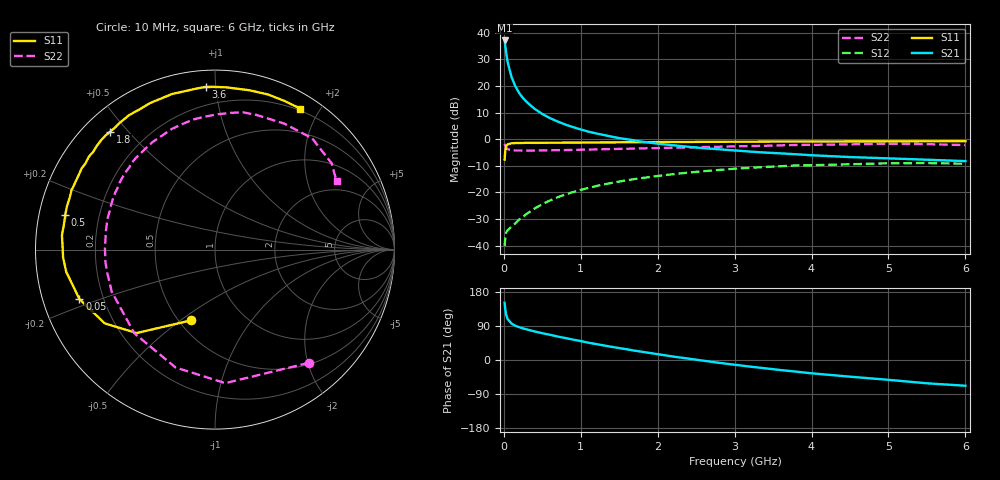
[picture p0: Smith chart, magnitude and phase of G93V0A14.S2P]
! SIEMENS Small Signal Semiconductors
! BFG235
! Si NPN RF Bipolar Junction Transistor in SOT223
! VCE = 3 V  IC = 140 mA
! Common Emitter S-Parameters:  July  1994
# GHz  S  MA  R  50
!  f  S11  S21  S12  S22
! GHz  MAG  ANG  MAG  ANG  MAG  ANG  MAG  ANG
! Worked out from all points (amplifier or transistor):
!   40 points, 10 MHz to 6 GHz, reference 50 ohm
!   highest |S21| = 37.1 dB at 10 MHz (marker M1)
!   |S21| within 3 dB of that: start of sweep to 23.17 MHz
!   unconditionally stable (mu >= 1): 443.8 MHz to 1.532 GHz
!   at 200 MHz: K = 0.81, MSG = 23.7 dB, |S12| = -30.1 dB
!   at 1.5 GHz: K = 1.00, MAG = 7.8 dB, |S12| = -15.9 dB
!   at 6 GHz: K = 0.91, MSG = 0.5 dB, |S12| = -9.2 dB
!   S11 on the Smith chart (normalised r, x): 10 MHz: 0.58, -0.55; 50 MHz: 0.11, -0.18; 500 MHz: 0.08, +0.11; 1.8 GHz: 0.08, +0.45; 3.6 GHz: 0.09, +0.94; 6 GHz: 0.18, +1.76
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0.01  0.4154 -108.5  71.63 150.7  0.0098 61.2  0.8197 -50.3
0.02  0.6378 -133.2  55.05 131.3  0.0147 46.4  0.7462 -85.6
0.03  0.739 -146.2  42.51 119.6  0.0177 39.7  0.6926 -108.5
0.05  0.804 -159.9  27.95 107.7  0.0195 32.5  0.6476 -134.0
0.1  0.8381 -171.5  14.66 96.2  0.0229 36.3  0.6213 -157.8
0.15  0.8475 -177.0  9.829 90.3  0.0264 43.0  0.614 -167.7
0.2  0.8485 180.0  7.353 86.6  0.0311 47.7  0.6144 -173.3
0.25  0.8518 177.0  5.924 83.2  0.0352 51.7  0.6126 -177.2
0.3  0.8565 174.7  4.947 80.6  0.04 54.3  0.6133 179.5
0.4  0.8532 170.5  3.725 75.3  0.05 57.0  0.6131 174.5
0.5  0.856 167.1  2.975 70.7  0.0603 57.8  0.6165 170.4
0.7  0.8598 160.4  2.146 61.9  0.0813 57.3  0.6234 163.1
0.9  0.8638 154.9  1.687 53.8  0.1017 54.3  0.6298 156.8
1.1  0.8698 148.6  1.386 45.6  0.1219 50.8  0.6397 150.6
1.4  0.8702 141.3  1.118 34.8  0.1507 44.7  0.6542 142.0
1.8  0.8787 131.6  0.897 21.6  0.1869 36.0  0.6745 130.9
2.2  0.889 122.6  0.77 9.1  0.2203 26.9  0.693 120.1
3.2  0.8982 101.4  0.586 -17.4  0.2905 3.6  0.7431 94.2
3.6  0.9081 93.3  0.542 -26.6  0.3114 -6.2  0.7671 83.4
4.5  0.9083 77.8  0.462 -44.0  0.3386 -25.7  0.8013 61.1
5.5  0.9145 64.7  0.412 -61.5  0.3564 -47.3  0.8085 36.5
6  0.918 58.8  0.388 -67.9  0.3467 -55.4  0.7771 29.4
